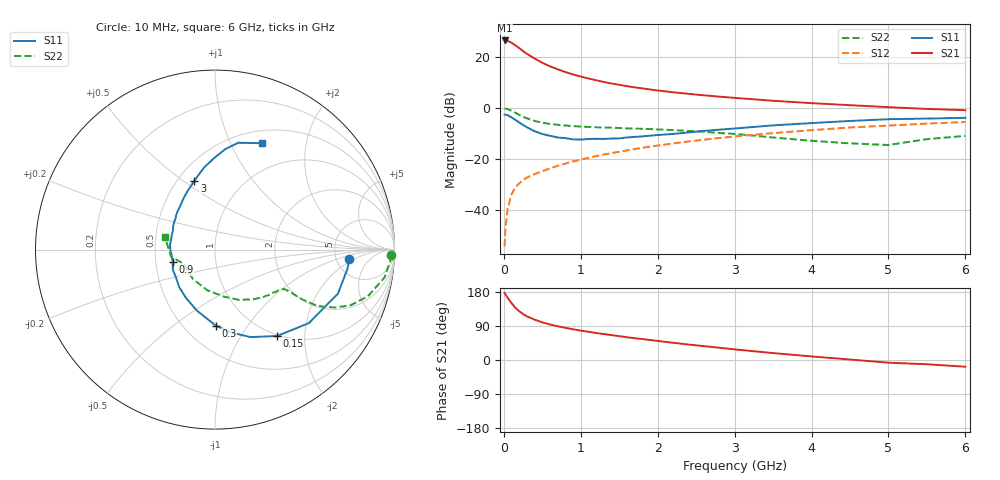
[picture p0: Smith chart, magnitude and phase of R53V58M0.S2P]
! SIEMENS Small Signal Semiconductors
! BFR183
! Si NPN RF Bipolar Junction Transistor in SOT23
! VCE = 3.5 V  IC = 8 mA
! Common Emitter S-Parameters:  May  1996
# GHz  S  MA  R  50
!  f  S11  S21  S12  S22
! GHz  MAG  ANG  MAG  ANG  MAG  ANG  MAG  ANG
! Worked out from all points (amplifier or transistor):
!   36 points, 10 MHz to 6 GHz, reference 50 ohm
!   highest |S21| = 26.5 dB at 10 MHz (marker M1)
!   |S21| within 3 dB of that: start of sweep to 200.9 MHz
!   unconditionally stable (mu >= 1): 855.2 MHz to 2.522 GHz
!   at 250 MHz: K = 0.55, MSG = 25.2 dB, |S12| = -28.1 dB
!   at 1.4 GHz: K = 1.06, MAG = 12.2 dB, |S12| = -17.6 dB
!   at 6 GHz: K = 0.89, MSG = 2.3 dB, |S12| = -5.4 dB
!   lowest NFmin = 1.30 dB at 450 MHz
!   S11 on the Smith chart (normalised r, x): 10 MHz: 6.61, -1.62; 150 MHz: 0.98, -1.46; 300 MHz: 0.70, -0.72; 900 MHz: 0.61, -0.09; 3 GHz: 0.60, +0.55; 6 GHz: 0.65, +1.32
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0.01  0.7504 -4.1  21.14 176.8  0.002 92.3  0.9832 -1.8
0.02  0.7459 -8.2  21.04 173.3  0.0043 84.1  0.9787 -3.7
0.05  0.7277 -19.7  20.84 164.1  0.0108 80.7  0.9577 -9.3
0.1  0.6641 -38.1  19.08 150.2  0.0205 73.2  0.8906 -17.0
0.15  0.5922 -54.4  16.96 137.7  0.0284 66.8  0.8144 -22.5
0.2  0.5261 -67.9  15 128.7  0.0339 63.6  0.7402 -25.8
0.25  0.4699 -79.2  13.09 121.2  0.0392 62.1  0.6792 -27.9
0.3  0.4237 -89.4  11.6 115.3  0.0438 61.0  0.6334 -29.0
0.4  0.3543 -106.7  9.366 106.5  0.0514 60.5  0.564 -29.7
0.5  0.3127 -121.5  7.735 99.3  0.0586 61.2  0.5184 -29.6
0.6  0.2885 -133.8  6.598 93.8  0.0665 61.6  0.4919 -29.4
0.7  0.2672 -144.5  5.766 89.0  0.0745 62.5  0.4732 -29.5
0.9  0.2456 -163.7  4.565 81.0  0.0909 63.3  0.4457 -29.7
1.1  0.2493 180.0  3.815 74.5  0.107 63.8  0.4302 -31.2
1.3  0.2504 167.3  3.259 68.5  0.1241 63.1  0.4186 -32.8
1.6  0.2677 150.5  2.697 60.1  0.1496 61.9  0.4035 -36.4
2.2  0.3134 127.7  2.049 45.5  0.2041 57.9  0.3738 -45.7
3  0.4009 106.7  1.593 28.0  0.2805 50.0  0.3147 -63.4
3.5  0.4612 97.6  1.397 18.3  0.3256 44.1  0.2674 -79.0
4.5  0.563 84.1  1.146 1.3  0.4199 31.9  0.2052 -126.9
5.5  0.6266 71.4  0.968 -11.2  0.4998 19.9  0.2483 -170.9
6  0.6478 66.2  0.913 -17.8  0.5369 12.1  0.2878 165.7
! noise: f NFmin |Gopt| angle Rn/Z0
0.45  1.3  0.17  43  0.21
0.9  1.35  0.21  115  0.2
1.8  2.05  0.33  -177  0.14
